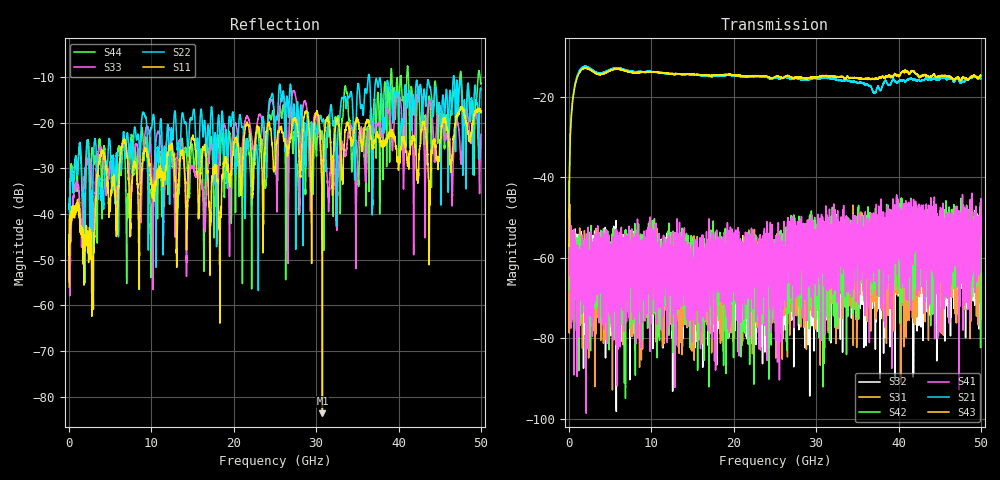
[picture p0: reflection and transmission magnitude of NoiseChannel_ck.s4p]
!Keysight Technologies,N5245A,MY49151038,A.10.65.06
!Date: Wednesday, June 07, 2023 11:03:22
!Correction: S11(Full 4 Port(1,2,3,4))
!S12(Full 4 Port(1,2,3,4))
!S13(Full 4 Port(1,2,3,4))
!S14(Full 4 Port(1,2,3,4))
!S21(Full 4 Port(1,2,3,4))
!S22(Full 4 Port(1,2,3,4))
!S23(Full 4 Port(1,2,3,4))
!S24(Full 4 Port(1,2,3,4))
!S31(Full 4 Port(1,2,3,4))
!S32(Full 4 Port(1,2,3,4))
!S33(Full 4 Port(1,2,3,4))
!S34(Full 4 Port(1,2,3,4))
!S41(Full 4 Port(1,2,3,4))
!S42(Full 4 Port(1,2,3,4))
!S43(Full 4 Port(1,2,3,4))
!S44(Full 4 Port(1,2,3,4))
!S4P File: Measurements: <S11,S12,S13,S14>,
!<S21,S22,S23,S24>,
!<S31,S32,S33,S34>,
!<S41,S42,S43,S44>:
# Hz S  RI  R 50
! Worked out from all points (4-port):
!   5000 points, 10 MHz to 50 GHz, reference 50 ohm
!   strongest paths, dB at 10 MHz, 12.51 GHz, 25.01 GHz, 37.51 GHz, 50 GHz:
!     S43: -57.1, -14.2, -15.0, -15.6, -14.8
!     S21: -46.5, -14.4, -15.2, -17.6, -15.4
!     S41: -41.7, -59.4, -63.7, -50.7, -54.4
!     S42: -41.0, -58.8, -57.9, -54.6, -54.5
!     S31: -46.9, -73.8, -65.8, -58.2, -50.7
!     S32: -42.9, -65.5, -58.7, -53.9, -53.9
!   lowest |S11| = -83.6 dB at 30.76 GHz (marker M1), VSWR 1.00, Z = 50 + j0.00562 ohm
!   |S11| at or under -10 dB: start of sweep to end of sweep
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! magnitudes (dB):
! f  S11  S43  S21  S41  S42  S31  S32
! 10 MHz  -56.0  -57.1  -46.5  -41.7  -41.0  -46.9  -42.9
! 480 MHz  -39.7  -20.6  -19.9  -61.2  -58.5  -61.0  -60.3
! 1.75 GHz  -48.1  -13.0  -12.6  -61.1  -62.6  -65.8  -65.5
! 6.68 GHz  -23.8  -13.5  -13.3  -68.0  -67.0  -70.4  -60.5
! 8.5 GHz  -49.6  -14.0  -13.8  -58.0  -56.8  -69.4  -57.1
! 30.76 GHz  -83.6  -14.8  -15.3  -56.0  -57.5  -56.8  -63.8
! 50 GHz  -17.5  -14.8  -15.4  -54.4  -54.5  -50.7  -53.9
